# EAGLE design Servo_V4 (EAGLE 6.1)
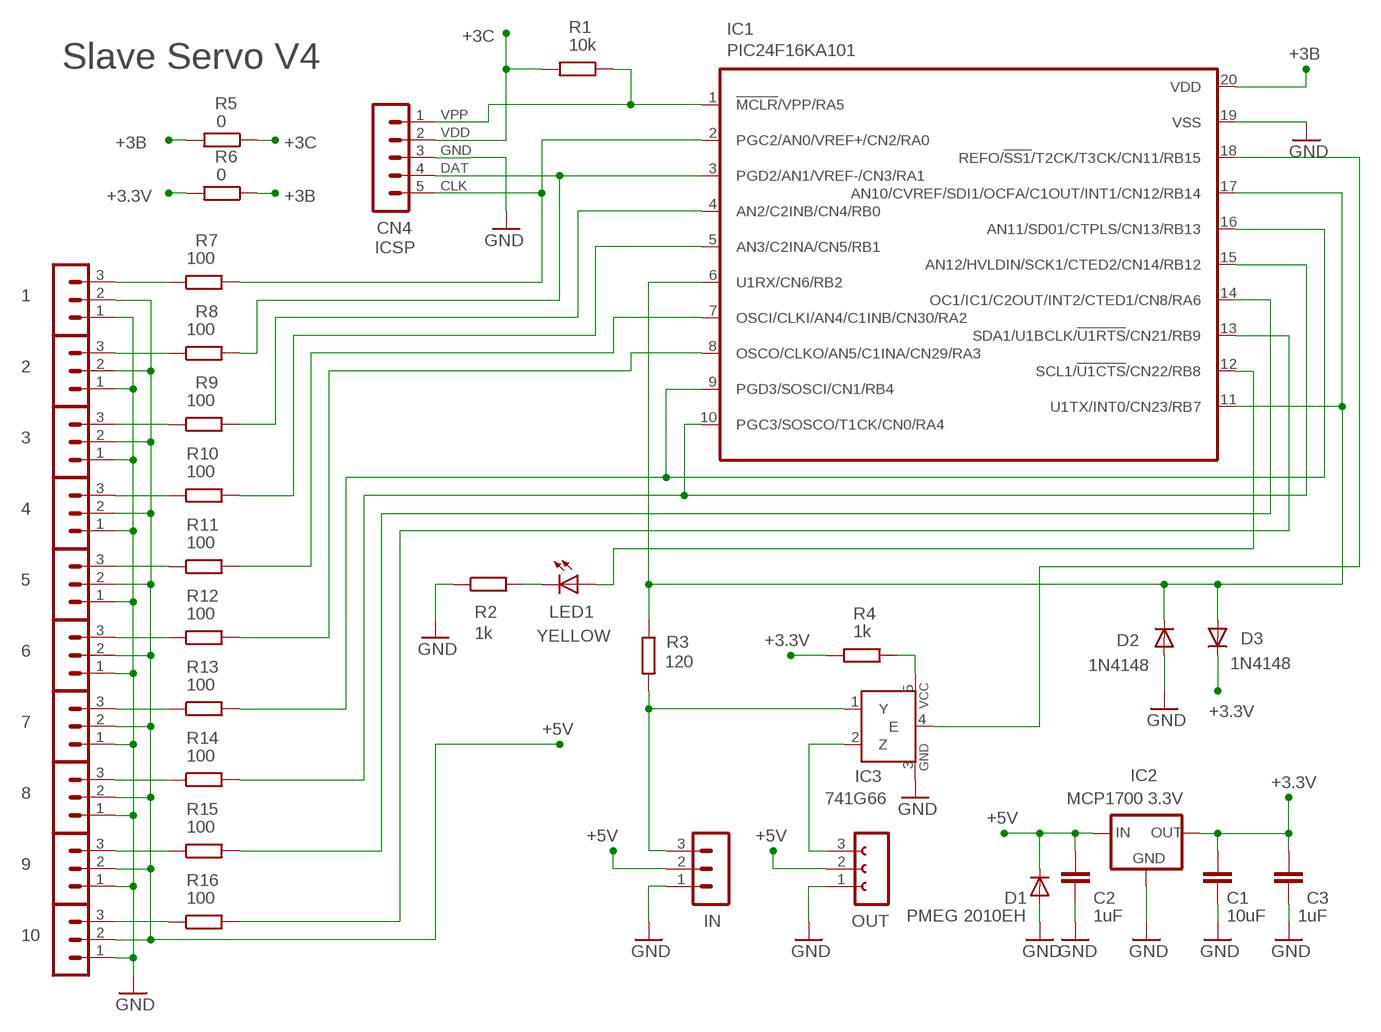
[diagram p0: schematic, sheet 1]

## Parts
1  OUT  MA03-1L1  [MA03-1_L1]
2  OUT  MA03-1L1  [MA03-1_L1]
3  OUT  MA03-1L1  [MA03-1_L1]
4  OUT  MA03-1L1  [MA03-1_L1]
5  OUT  MA03-1L1  [MA03-1_L1]
6  OUT  MA03-1L1  [MA03-1_L1]
7  OUT  MA03-1L1  [MA03-1_L1]
8  OUT  MA03-1L1  [MA03-1_L1]
9  OUT  MA03-1L1  [MA03-1_L1]
10  OUT  MA03-1L1  [MA03-1_L1]
C1  10uF  C-EUC0805  [C0805]
C2  1uF  C-EUC0603  [C0603]
C3  1uF  C-EUC0603  [C0603]
CN4  ICSP  MA05-1  [MA05-1]
D1  PMEG 2010EH  DIODE-SOD123-B  [SOD123-B]
D2  1N4148  DIODE-SOD123-B  [SOD123-B]
D3  1N4148  DIODE-SOD123-B  [SOD123-B]
IC1  PIC24F16KA101  PIC24F04KA201SOIC  [SOIC20_S]
IC2  MCP1700 3.3V  MCP1700SOT23  [SOT23]
IC3  741G66  741G66DBV  [SOT23-5]
IN  MA03-1N  [MA03-1]
LED1  YELLOW  LED3MM_F  [LED3MM]
OUT  FE03-1"  [FE03-1]
R1  10k  R-EU_R0805  [R0805]
R2  1k  R-EU_R1206_L  [R1206_L]
R3  120  R-EU_R0805  [R0805]
R4  1k  R-EU_R0603  [R0603]
R5  0  R-EU_R1206_L  [R1206_L]
R6  0  R-EU_R1206_L  [R1206_L]
R7  100  R-EU_R0603  [R0603]
R8  100  R-EU_R0603  [R0603]
R9  100  R-EU_R0603  [R0603]
R10  100  R-EU_R0603  [R0603]
R11  100  R-EU_R0603  [R0603]
R12  100  R-EU_R0603  [R0603]
R13  100  R-EU_R0603  [R0603]
R14  100  R-EU_R0603  [R0603]
R15  100  R-EU_R0603  [R0603]
R16  100  R-EU_R0603  [R0603]

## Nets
+3.3V: C1.1 C3.1 D3.C IC2.2(OUT) R4.1 R6.2
+3B: IC1.20(VDD) R5.2 R6.1
+3C: CN4.2 R1.2 R5.1
+5V: 1.2 2.2 3.2 4.2 5.2 6.2 7.2 8.2 9.2 10.2 C2.1 D1.C IC2.3(IN) IN.2 OUT.2
GND: 1.1 2.1 3.1 4.1 5.1 6.1 7.1 8.1 9.1 10.1 C1.2 C2.2 C3.2 CN4.3 D1.A D2.A IC1.19(VSS) IC2.1(GND) IC3.3(GND) IN.1 OUT.1 R2.1
N$1: IC1.18(REFO/!SS1!/T2CK/T3CK/CN11/RB15) IC3.4(E)
N$2: IC1.9(PGD3/SOSCI/CN1/RB4) IC1.16(AN11/SD01/CTPLS/CN13/RB13) R13.2
N$3: D2.C D3.A IC1.6(U1RX/CN6/RB2) IC1.11(U1TX/INT0/CN23/RB7) IC1.17(AN10/CVREF/SDI1/OCFA/C1OUT/INT1/CN12/RB14) R3.1
N$4: CN4.1 IC1.1(!MCLR!/VPP/RA5) R1.1
N$5: IC3.5(VCC) R4.2
N$6: LED1.K(C) R2.2
N$7: IC1.7(OSCI/CLKI/AN4/C1INB/CN30/RA2) R11.2
N$8: IC1.8(OSCO/CLKO/AN5/C1INA/CN29/RA3) R12.2
N$9: IC1.5(AN3/C2INA/CN5/RB1) R10.2
N$10: 1.3 R7.1
N$11: IC1.10(PGC3/SOSCO/T1CK/CN0/RA4) IC1.15(AN12/HVLDIN/SCK1/CTED2/CN14/RB12) R14.2
N$12: IC1.12(SCL1/!U1CTS!/CN22/RB8) LED1.A
N$13: IC1.13(SDA1/U1BCLK/!U1RTS!/CN21/RB9) R16.2
N$14: 2.3 R8.1
N$15: IC3.2(Z) OUT.3
N$16: IC3.1(Y) IN.3 R3.2
N$17: IC1.14(OC1/IC1/C2OUT/INT2/CTED1/CN8/RA6) R15.2
N$18: 3.3 R9.1
N$19: 4.3 R10.1
N$20: CN4.5 IC1.2(PGC2/AN0/VREF+/CN2/RA0) R7.2
N$21: CN4.4 IC1.3(PGD2/AN1/VREF-/CN3/RA1) R8.2
N$22: IC1.4(AN2/C2INB/CN4/RB0) R9.2
N$23: 5.3 R11.1
N$24: 6.3 R12.1
N$25: 7.3 R13.1
N$26: 8.3 R14.1
N$27: 9.3 R15.1
N$28: 10.3 R16.1

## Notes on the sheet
- Slave Servo V4

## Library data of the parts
1-10 IN = 03-con-lstb-M:MA03-1: PIN HEADER
C1-C3 = 00-LIVIO:C-EU: CAPACITOR, European symbol
CN4 = 03-con-lstb-M:MA05-1: PIN HEADER; CLK: CLK; DAT: DAT; GND: GND; VDD: VDD; VPP: VPP
D1-D3 = 00-LIVIO:DIODE-: DIODE
IC1 = 00-LIVIO:PIC24F04KA201
IC2 = 00-LIVIO:MCP1700: Linear regulator Quescient courrent 1.8uA Input 2.3v to 6v Output 1.2v 1.8v 2.5v 3.0v 3.3v 5.0v
IC3 = 00-LIVIO:74*1G66: Single Analog / Bilateral Switch Source: http://www.semiconductors.philips.com/acrobat_download/datasheets/74HC_HCT1G66_3.pdf
LED1 = 00-LIVIO:LED: LEDS
OUT = 02-con-lsta-F:FE03-1: FEMALE HEADER
R1-R16 = 00-LIVIO:R-EU_: RESISTOR, European symbol

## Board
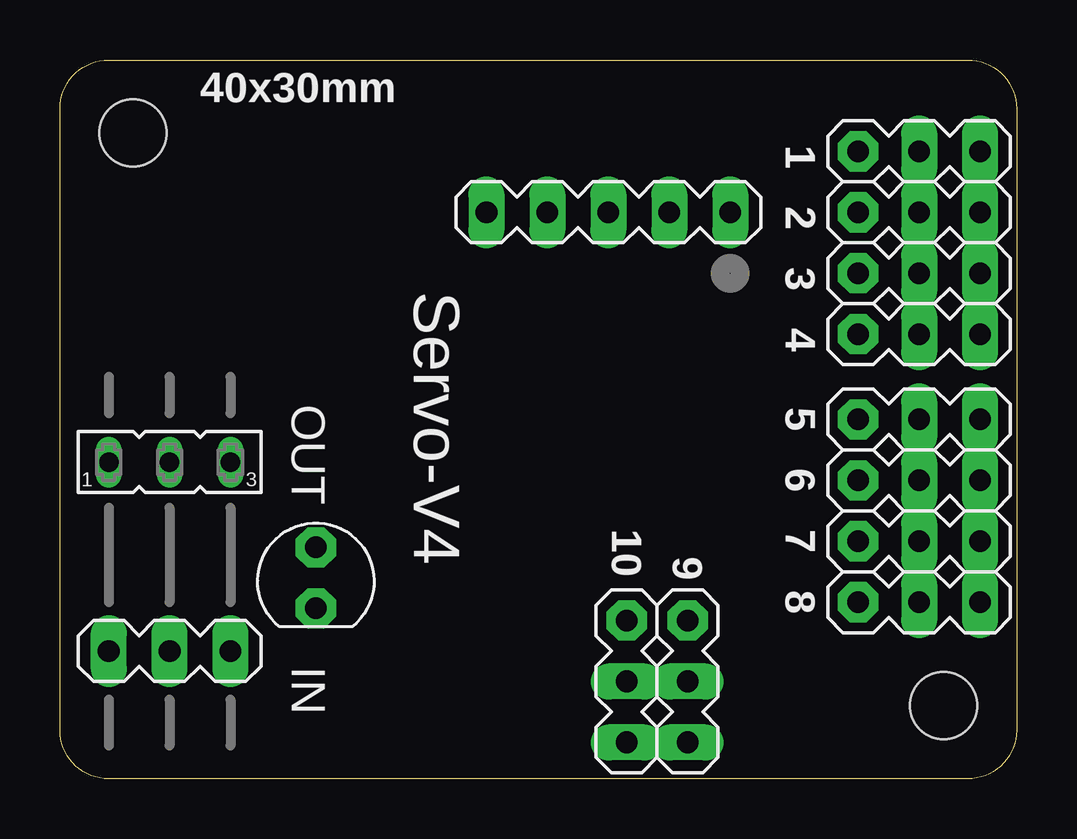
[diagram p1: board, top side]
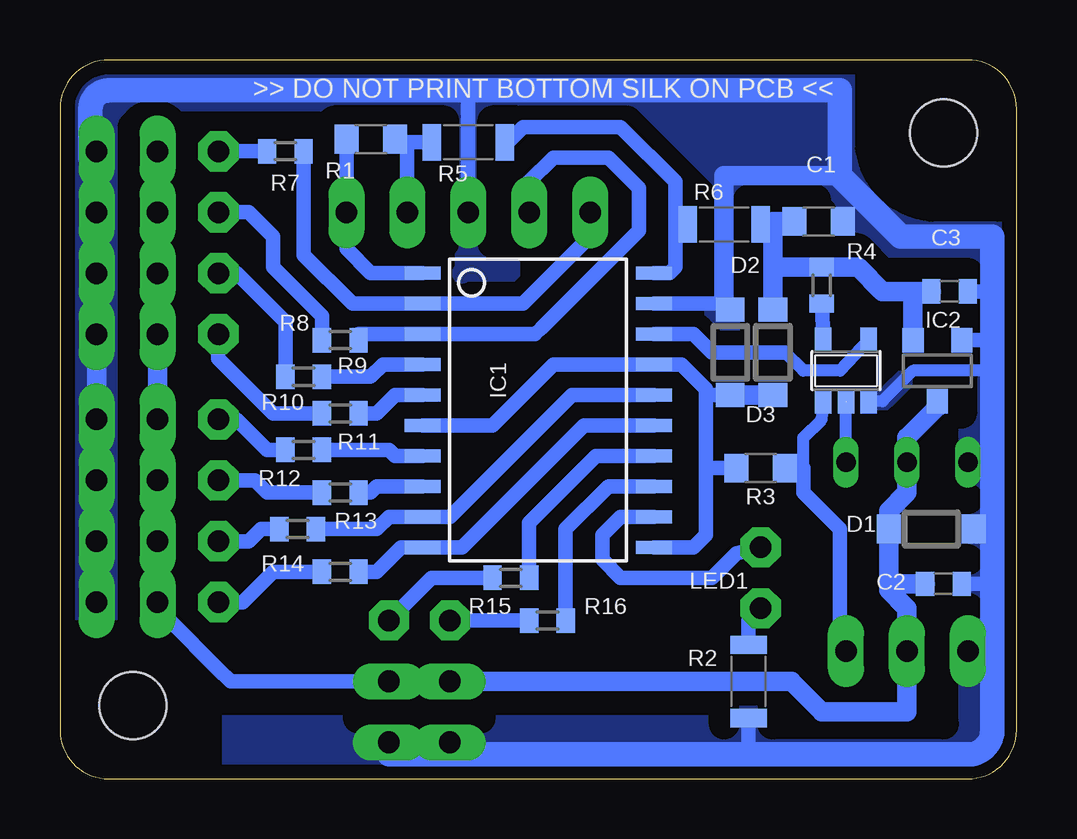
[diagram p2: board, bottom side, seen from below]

Size 39.88 x 29.97 mm. Coordinates in mm from the lower left corner, seen from the top.
Outline: 37.85,0 2.03,0 arc-90 0,2.03 0,27.94 arc-90 2.03,29.97 37.85,29.97 arc-90 39.88,27.94 39.88,2.03 arc-90 37.85,0
Copper layers (1*16): Top 0.035mm / dielectric 1.5mm / Bottom 0.035mm
Design rules: minimum track width 10mil, minimum drill 19mil, track to track 19mil, track to pad 19mil, pad to pad 19mil, via to via 19mil, smd to smd 19mil, copper to edge 19mil, drill to drill 8mil, minimum pad ring 5mil, minimum via ring 8mil, stop-mask expansion 4mil, vias tented up to drill 0mil, thermal gap 29mil
Holes 2.8 mm at 3.05,26.92 36.83,3.05
bRestrict: 46 lines

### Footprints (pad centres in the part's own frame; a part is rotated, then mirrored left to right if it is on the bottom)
MA03-1_L1 = drill 0.9 pad 1.5 long: 1 -2.54,0; 2 0,0 | drill 0.9 pad 1.676 octagon: 3 2.54,0
C0805 = smd 1 x 1.2: 1 -1.016,0; 2 1.016,0
C0603 = smd 0.762 x 1.016: 1 -0.762,0; 2 0.762,0
MA05-1 = drill 0.9 pad 1.5 long: 1 -5.08,0; 2 -2.54,0; 3 0,0; 4 2.54,0; 5 5.08,0
SOD123-B = smd 1 x 1.2: A 1.778,0; C -1.778,0
SOIC20_S = smd 0.55 x 1.5: 1 -5.715,-4.826; 2 -4.445,-4.826; 3 -3.175,-4.826; 4 -1.905,-4.826; 5 -0.635,-4.826; 6 0.635,-4.826; 7 1.905,-4.826; 8 3.175,-4.826; 9 4.445,-4.826; 10 5.715,-4.826; 11 5.715,4.826; 12 4.445,4.826; 13 3.175,4.826; 14 1.905,4.826; 15 0.635,4.826; 16 -0.635,4.826; 17 -1.905,4.826; 18 -3.175,4.826; 19 -4.445,4.826; 20 -5.715,4.826
SOT23 = smd 0.889 x 1.016: 1 -1.016,-1.27; 2 1.016,-1.27; 3 0,1.27
SOT23-5 = smd 0.69 x 0.99: 1 -0.95,-1.29; 2 0,-1.29; 3 0.95,-1.29; 4 0.95,1.3; 5 -0.95,1.3
MA03-1 = drill 0.9 pad 1.5 long: 1 -2.54,0; 2 0,0; 3 2.54,0
LED3MM = drill 0.9 pad 1.676 octagon: A -1.27,0; K 1.27,0
FE03-1 = drill 0.813 long: 1 -2.54,0; 2 0,0; 3 2.54,0
R0805 = smd 1 x 1.2: 1 -1.016,0; 2 1.016,0
R1206_L = smd 0.762 x 1.524: 1 -1.524,0; 2 1.524,0
R0603 = smd 0.762 x 1.016: 1 -0.762,0; 2 0.762,0

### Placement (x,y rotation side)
1  35.81,26.16 180 top
2  35.81,23.62 180 top
3  35.81,21.08 180 top
4  35.81,18.54 180 top
5  35.81,14.99 180 top
6  35.81,12.45 180 top
7  35.81,9.91 180 top
8  35.81,7.37 180 top
9  26.16,4.06 90 top
10  23.62,4.06 90 top
C1  8.26,23.24 0 bottom
C2  3.05,8.13 0 bottom
C3  2.79,20.32 0 bottom
CN4  22.86,23.62 180 top
D1  3.56,10.41 0 bottom
D2  11.94,17.78 90 bottom
D3  10.16,17.78 270 bottom
IC1  19.94,15.37 270 bottom
IC2  3.3,17.02 180 bottom
IC3  7.11,17.02 0 bottom
IN  4.57,5.33 0 top
LED1  10.67,8.38 270 top
OUT  4.57,13.21 0 top
R1  26.92,26.67 0 bottom
R2  11.18,4.06 90 bottom
R3  10.67,12.95 0 bottom
R4  8.13,20.57 270 bottom
R5  22.86,26.54 0 bottom
R6  12.19,23.11 0 bottom
R7  30.48,26.16 0 bottom
R8  28.19,18.29 0 bottom
R9  29.72,16.76 0 bottom
R10  28.19,15.24 0 bottom
R11  29.72,13.72 0 bottom
R12  28.19,11.94 0 bottom
R13  29.97,10.41 0 bottom
R14  28.19,8.64 0 bottom
R15  21.08,8.38 0 bottom
R16  19.56,6.6 0 bottom

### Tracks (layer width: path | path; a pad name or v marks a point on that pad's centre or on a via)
+3.3V
  Bottom 0.61: 4.32,20.32 5.59,20.32
  Bottom 0.813: IC2.2 4.32,20.32 | C3.1 5.59,20.32 6.6,21.34 R4.1 10.16,21.34 | D3.C 10.16,21.34 | 10.16,21.34 10.16,23.11 | 10.16,23.11 R6.2 | C1.1 10.16,23.24 10.16,23.11
+3B
  Bottom 0.61: R5.2 21.21,26.54 20.57,27.18 16.51,27.18 14.22,24.89 14.22,23.11 | 14.22,23.11 14.22,21.34 14.48,21.08 IC1.20 | R6.1 14.22,23.11
+3C
  Bottom 0.61: CN4.2 25.4,26.54 | 25.4,26.54 R5.1 | 25.4,26.54 25.91,26.54 R1.2
+5V
  Bottom 0.61: 8.2 35.81,6.6 35.31,6.6 33.27,4.57 32.77,4.06 9.2
  Bottom 0.813: 1.2 2.2 3.2 4.2 5.2 6.2 7.2 8.2 | 9.2 10.2 22.61,4.06 17.78,4.06 | 5.33,7.87 D1.C 5.33,11.18 4.57,11.94 OUT.2 4.57,14.22 3.3,15.49 IC2.3 | 5.33,7.87 5.33,8.13 C2.1 | 5.33,7.87 4.57,7.11 IN.2 4.57,2.79 8.13,2.79 9.4,4.06 17.53,4.06 | 17.53,4.06 17.78,4.06 | 17.78,4.06 17.53,4.06 | 17.53,4.06 17.78,4.06
GND
  Bottom 0.508: IC3.3 5.59,15.75 4.32,17.02 1.02,17.02
  Bottom 0.61: 1.02,18.29 IC2.1 | 1.02,10.41 D1.A | IC1.19 12.19,19.81 11.94,19.81 D2.A | 1.02,20.32 C3.2 | 1.02,8.13 C2.2 | CN4.3 22.86,28.7 | R2.1 11.18,1.02
  Bottom 0.813: 1.1 2.1 3.1 4.1 5.1 6.1 7.1 8.1 | 7.37,25.15 12.19,25.15 12.19,19.81 D2.A | OUT.1 1.02,13.21 | IN.1 1.02,5.33
  Bottom 1.016: 23.62,1.02 10.1 23.62,1.02 | 23.62,1.02 26.16,1.02 9.1 | 23.62,1.02 11.18,1.02 2.03,1.02 arc-90 1.02,2.03 1.02,2.29 1.02,5.33 1.02,8.13 1.02,10.41 1.02,13.21 1.02,17.02 1.02,18.29 1.02,18.8 1.02,20.32 1.02,22.61 4.83,22.61 7.37,25.15 7.37,28.7 22.86,28.7 37.85,28.7 arc-90 38.61,27.94 38.61,27.69 38.61,25.91 1.1
  pour Bottom (isolate 0.6, no thermals): -1,-1 40.88,-1 40.88,30.97 -1,30.97
N$1
  Bottom 0.508: IC3.4 7.37,17.02 8.89,17.02 9.65,17.78
  Bottom 0.61: 9.65,17.78 12.7,17.78 13.46,18.54 IC1.18
N$2
  Bottom 0.61: IC1.16 18.54,16 23.62,10.92 IC1.9 26.16,10.92 26.67,10.41 R13.2
N$3
  Bottom 0.61: 12.95,12.95 R3.1 | 12.95,12.95 12.95,10.16 13.46,9.65 IC1.11 | 12.95,16 D2.C 12.95,16 | 12.95,12.95 12.95,16 | IC1.6 21.84,14.73 19.3,17.27 IC1.17 13.97,17.27 12.95,16.26 12.95,16
  Bottom 0.813: D2.C D3.A
N$4
  Bottom 0.61: IC1.1 26.92,21.08 27.94,22.1 CN4.1 R1.1
N$5
  Bottom 0.61: IC3.5 R4.2
N$6
  Bottom 0.61: LED1.K 11.18,6.6 R2.2
N$7
  Bottom 0.61: IC1.7 25.91,13.46 26.16,13.72 R11.2
N$8
  Bottom 0.61: IC1.8 26.67,12.19 26.92,11.94 R12.2
N$9
  Bottom 0.61: IC1.5 25.91,16 26.67,15.24 R10.2
N$10
  Bottom 0.61: R7.1 1.3
N$11
  Bottom 0.61: IC1.15 18.03,14.73 23.11,9.65 IC1.10 25.65,9.65 26.67,8.64 R14.2
N$12
  Bottom 0.61: IC1.12 16.51,10.92 17.27,10.16 17.27,9.14 16.51,8.38 12.7,8.38 11.68,9.4 LED1.A
N$13
  Bottom 0.61: IC1.13 17.02,12.19 18.8,10.41 R16.2
N$14
  Bottom 0.61: 2.3 32,23.62 30.99,22.61 30.99,21.34 28.96,19.3 R8.1
N$15
  Bottom 0.508: OUT.3 IC3.2
N$16
  Bottom 0.508: 8.89,12.95 8.89,14.22 8.13,14.99 IC3.1
  Bottom 0.61: R3.2 8.89,12.95 8.89,11.94 7.37,10.41 7.37,6.35 7.11,6.1 IN.3
N$17
  Bottom 0.61: IC1.14 17.53,13.46 20.32,10.67 R15.2
N$18
  Bottom 0.61: 3.3 32.51,21.08 30.48,19.05 R9.1
N$19
  Bottom 0.61: R10.1 30.99,15.24 33.27,17.53 4.3
N$20
  Bottom 0.61: CN4.5 17.78,22.61 20.57,19.81 IC1.2 27.69,19.81 29.72,21.84 R7.2
N$21
  Bottom 0.61: R8.2 27.43,18.54 IC1.3 20.07,18.54 19.81,18.8 15.75,22.86 15.75,24.13 15.75,24.64 17.02,25.91 19.3,25.91 20.32,24.89 CN4.4
N$22
  Bottom 0.61: IC1.4 26.42,17.27 26.92,16.76 R9.2
N$23
  Bottom 0.61: R11.1 31.24,13.72 32.51,14.99 5.3
N$24
  Bottom 0.61: R12.1 31.24,11.94 31.75,12.45 6.3
N$25
  Bottom 0.61: R13.1 31.5,10.41 32,9.91 7.3
N$26
  Bottom 0.61: R14.1 30.99,8.64 32.26,7.37 8.3
N$27
  Bottom 0.61: R15.1 24.38,8.38 9.3
N$28
  Bottom 0.61: 10.3 R16.1
N$29
  pour Bottom (no thermals): 22.73,21.08 arc180 23.5,21.08 arc180

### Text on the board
tNames: 40x30mm | Servo-V4
bNames: >> DO NOT PRINT BOTTOM SILK ON PCB <<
